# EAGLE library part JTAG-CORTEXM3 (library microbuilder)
Serial Wire (SW-DP) Connector This standard 0.05" 10-pin connector is for use with the Cortex M0/M3's native SWD (serial wire debugger) interface (SW-DP). Some boards support a 20-pin combined JTAG+SWD connector (SWJ-DP), such as the LPC1700 family, but many smaller devices only work with SWD which typically use the smaller 10-pin SW-DP connecter (the LPC1300 family, for example, only supports SWD). 2x05 1.27mm/0.05" Connector: This is the standard SMT connector defined by ARM for all Cortex devices, and should be used in most situations and for forward-compatibility since any new devices coming to market will likely use this connector. MOLEX 10 Pin 0.1" Connector: This 0.1" 10 pin connector has the same pin layout as the standard 0.05" connector, but is easier to work with if you are using standard jumper wires or custom cables to connect your SWD hardware. MOLEX 20 Pin 0.1" Connector: This 0.1" 20 pin connector is the same model used for ARM7/ARM9 JTAG debuggers, but is connected to match the pins on the Segger J-Link for ARM (which supports both JTAG and SWD debugging). See the following document from ARM for more information on Cortex M3 Debug Connectors: http://infocenter.arm.com/help/topic/com.arm.doc.faqs/attached/13634/cortex_debug_connectors.pdf And the following page for an overview with images of the different connector types: http://www.keil.com/peripherals/coresight/connectors.asp
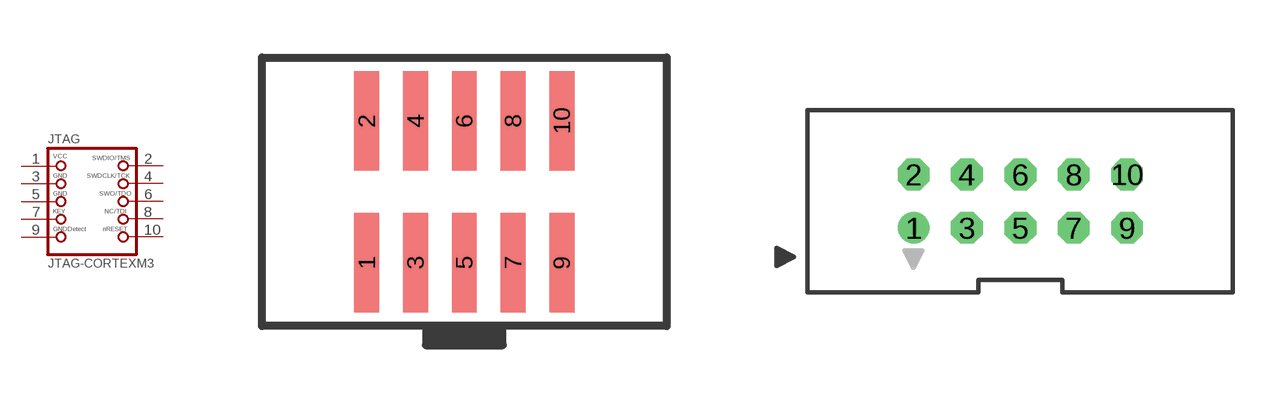
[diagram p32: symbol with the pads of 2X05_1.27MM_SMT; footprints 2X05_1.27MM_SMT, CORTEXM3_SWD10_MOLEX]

Designator prefix JTAG

## JTAG-CORTEXM3  [2X05_1.27MM_SMT]
1  1  pas
2  2  pas
3  3  pas
4  4  pas
5  5  pas
6  6  pas
7  7  pas
8  8  pas
9  9  pas
10  10  pas

## JTAG-CORTEXM3MOLEX  [CORTEXM3_SWD10_MOLEX]
Pads as for 2X05_1.27MM_SMT

## JTAG-CORTEXM3MOLEX20  [JTAG-ARM]
1  1  pas
4  3  pas
6  5  pas
7  2  pas
8  9  pas
9  4  pas
10  7  pas
13  6  pas
15  10  pas
17  8  pas

## Footprint 2X05_1.27MM_SMT (pad centres in mm)
2x05 1.27mm Headers SMT (2.0mm Height) 4UConnector: 16846
smd 0.65 x 2.6: 1 -2.54,-1.85; 2 -2.54,1.85; 3 -1.27,-1.85; 4 -1.27,1.85; 5 0,-1.85; 6 0,1.85; 7 1.27,-1.85; 8 1.27,1.85; 9 2.54,-1.85; 10 2.54,1.85

## Footprint CORTEXM3_SWD10_MOLEX (pad centres in mm)
10 Pin SWD Connector (Cortex M3) Note: Small tRestrict polygon's were added to the ground pads to improve solderability when this part is used in combination with a ground pour. By default, Eagle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
drill 1: 1 -5.08,-1.27
drill 1 octagon: 2 -5.08,1.27; 3 -2.54,-1.27; 4 -2.54,1.27; 5 0,-1.27; 6 0,1.27; 7 2.54,-1.27; 8 2.54,1.27; 9 5.08,-1.27; 10 5.08,1.27

## Footprint JTAG-ARM (pad centres in mm)
20 Pin JTAG Connector (ARM7, ARM9)
drill 1: 1 -11.43,-1.27
drill 1 octagon: 2 -11.43,1.27; 3 -8.89,-1.27; 4 -8.89,1.27; 5 -6.35,-1.27; 6 -6.35,1.27; 7 -3.81,-1.27; 8 -3.81,1.27; 9 -1.27,-1.27; 10 -1.27,1.27; 11 1.27,-1.27; 12 1.27,1.27; 13 3.81,-1.27; 14 3.81,1.27; 15 6.35,-1.27; 16 6.35,1.27; 17 8.89,-1.27; 18 8.89,1.27; 19 11.43,-1.27; 20 11.43,1.27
